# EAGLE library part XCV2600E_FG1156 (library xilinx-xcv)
xcv2600e_fg1156 edit this description Auto generated by make-symbol-device-package-bsdl.ulp Rev. 26 Source: xcv2600e_fg1156.bsd
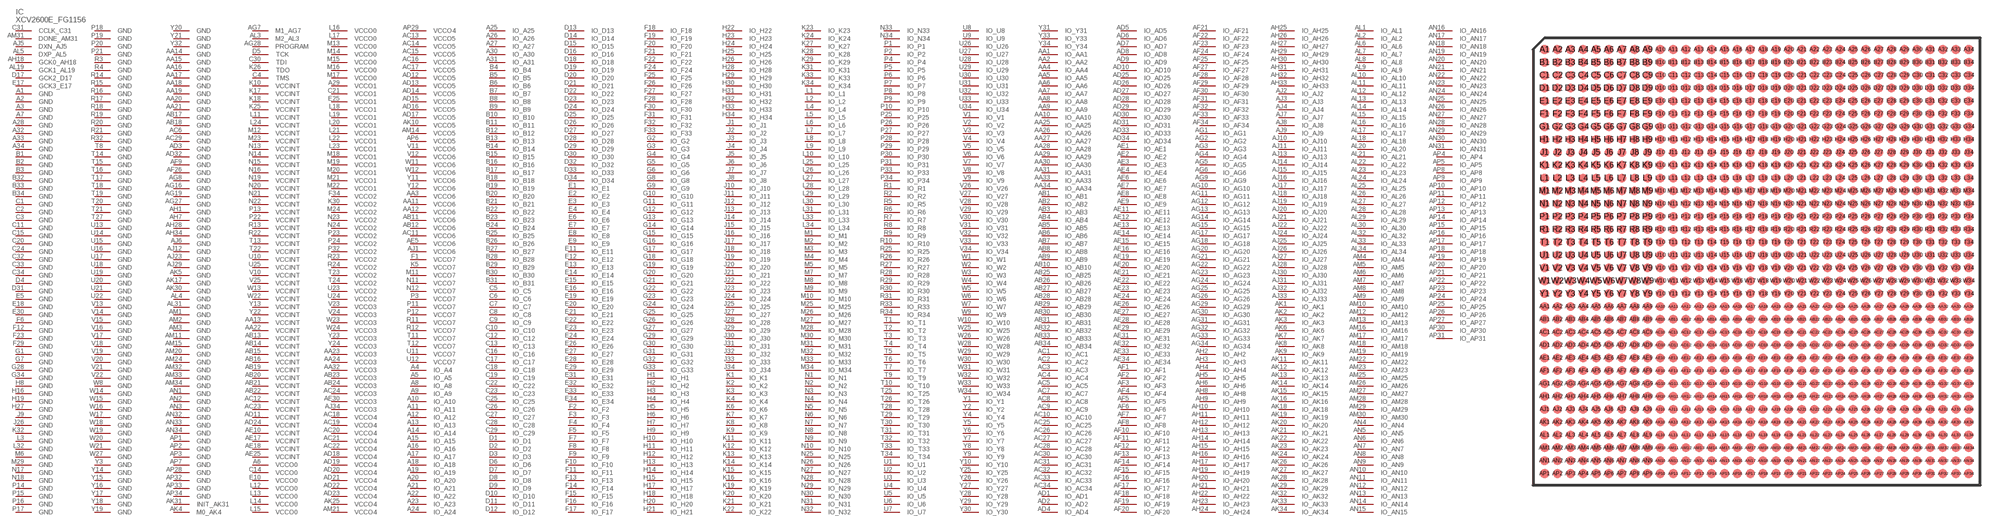
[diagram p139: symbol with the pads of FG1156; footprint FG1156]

Designator prefix IC

## XCV2600E_FG1156 (OC_FARNELL: unknown; OC_NEWARK: unknown)  [FG1156]
A1  GND  pwr
A2  GND  pwr
A3  GND  pwr
A4  IO_A4
A5  IO_A5
A6  VCCO0  pwr
A7  GND  pwr
A8  IO_A8
A9  IO_A9
A10  IO_A10
A11  IO_A11
A12  IO_A12
A13  IO_A13
A14  IO_A14
A15  IO_A15
A16  IO_A16
A17  IO_A17
A18  IO_A18
A19  IO_A19
A20  IO_A20
A21  IO_A21
A22  IO_A22
A23  IO_A23
A24  IO_A24
A25  IO_A25
A26  IO_A26
A27  IO_A27
A28  GND  pwr
A29  VCCO1  pwr
A30  IO_A30
A31  IO_A31
A32  GND  pwr
A33  GND  pwr
A34  GND  pwr
AA1  IO_AA1
AA2  IO_AA2
AA3  VCCO6  pwr
AA4  IO_AA4
AA5  IO_AA5
AA6  IO_AA6
AA7  IO_AA7
AA8  IO_AA8
AA9  IO_AA9
AA10  IO_AA10
AA11  VCCO6  pwr
AA12  VCCO6  pwr
AA13  VCCINT  pwr
AA14  GND  pwr
AA15  GND  pwr
AA16  GND  pwr
AA17  GND  pwr
AA18  GND  pwr
AA19  GND  pwr
AA20  GND  pwr
AA21  GND  pwr
AA22  VCCINT  pwr
AA23  VCCO3  pwr
AA24  VCCO3  pwr
AA25  IO_AA25
AA26  IO_AA26
AA27  IO_AA27
AA28  IO_AA28
AA29  IO_AA29
AA30  IO_AA30
AA31  IO_AA31
AA32  VCCO3  pwr
AA33  IO_AA33
AA34  IO_AA34
AB1  IO_AB1
AB2  IO_AB2
AB3  IO_AB3
AB4  IO_AB4
AB5  IO_AB5
AB6  IO_AB6
AB7  IO_AB7
AB8  IO_AB8
AB9  IO_AB9
AB10  IO_AB10
AB11  VCCO6  pwr
AB12  VCCO6  pwr
AB13  VCCINT  pwr
AB14  VCCINT  pwr
AB15  VCCINT  pwr
AB16  VCCINT  pwr
AB17  GND  pwr
AB18  GND  pwr
AB19  VCCINT  pwr
AB20  VCCINT  pwr
AB21  VCCINT  pwr
AB22  VCCINT  pwr
AB23  VCCO3  pwr
AB24  VCCO3  pwr
AB25  IO_AB25
AB26  IO_AB26
AB27  IO_AB27
AB28  IO_AB28
AB29  IO_AB29
AB30  IO_AB30
AB31  IO_AB31
AB32  IO_AB32
AB33  IO_AB33
AB34  IO_AB34
AC1  IO_AC1
AC2  IO_AC2
AC3  IO_AC3
AC4  IO_AC4
AC5  IO_AC5
AC6  GND  pwr
AC7  IO_AC7
AC8  IO_AC8
AC9  IO_AC9
AC10  IO_AC10
AC11  VCCO6  pwr
AC12  VCCINT  pwr
AC13  VCCO5  pwr
AC14  VCCO5  pwr
AC15  VCCO5  pwr
AC16  VCCO5  pwr
AC17  VCCO5  pwr
AC18  VCCO4  pwr
AC19  VCCO4  pwr
AC20  VCCO4  pwr
AC21  VCCO4  pwr
AC22  VCCO4  pwr
AC23  VCCINT  pwr
AC24  VCCO3  pwr
AC25  IO_AC25
AC26  IO_AC26
AC27  IO_AC27
AC28  IO_AC28
AC29  GND  pwr
AC30  IO_AC30
AC31  IO_AC31
AC32  IO_AC32
AC33  IO_AC33
AC34  IO_AC34
AD1  IO_AD1
AD2  IO_AD2
AD3  GND  pwr
AD4  IO_AD4
AD5  IO_AD5
AD6  IO_AD6
AD7  IO_AD7
AD8  IO_AD8
AD9  IO_AD9
AD10  IO_AD10
AD11  VCCINT  pwr
AD12  VCCO5  pwr
AD13  VCCO5  pwr
AD14  VCCO5  pwr
AD15  VCCO5  pwr
AD16  VCCO5  pwr
AD17  VCCO5  pwr
AD18  VCCO4  pwr
AD19  VCCO4  pwr
AD20  VCCO4  pwr
AD21  VCCO4  pwr
AD22  VCCO4  pwr
AD23  VCCO4  pwr
AD24  VCCINT  pwr
AD25  IO_AD25
AD26  IO_AD26
AD27  IO_AD27
AD28  IO_AD28
AD29  IO_AD29
AD30  IO_AD30
AD31  IO_AD31
AD32  GND  pwr
AD33  IO_AD33
AD34  IO_AD34
AE1  IO_AE1
AE2  IO_AE2
AE3  IO_AE3
AE4  IO_AE4
AE5  VCCO6  pwr
AE6  IO_AE6
AE7  IO_AE7
AE8  IO_AE8
AE9  IO_AE9
AE10  VCCINT  pwr
AE11  IO_AE11
AE12  IO_AE12
AE13  IO_AE13
AE14  IO_AE14
AE15  IO_AE15
AE16  IO_AE16
AE17  VCCINT  pwr
AE18  VCCINT  pwr
AE19  IO_AE19
AE20  IO_AE20
AE21  IO_AE21
AE22  IO_AE22
AE23  IO_AE23
AE24  IO_AE24
AE25  VCCINT  pwr
AE26  IO_AE26
AE27  IO_AE27
AE28  IO_AE28
AE29  IO_AE29
AE30  VCCO3  pwr
AE31  IO_AE31
AE32  IO_AE32
AE33  IO_AE33
AE34  IO_AE34
AF1  IO_AF1
AF2  IO_AF2
AF3  IO_AF3
AF4  IO_AF4
AF5  IO_AF5
AF6  IO_AF6
AF7  IO_AF7
AF8  IO_AF8
AF9  GND  pwr
AF10  IO_AF10
AF11  IO_AF11
AF12  IO_AF12
AF13  IO_AF13
AF14  IO_AF14
AF15  IO_AF15
AF16  IO_AF16
AF17  IO_AF17
AF18  IO_AF18
AF19  IO_AF19
AF20  IO_AF20
AF21  IO_AF21
AF22  IO_AF22
AF23  IO_AF23
AF24  IO_AF24
AF25  IO_AF25
AF26  GND  pwr
AF27  IO_AF27
AF28  IO_AF28
AF29  IO_AF29
AF30  IO_AF30
AF31  IO_AF31
AF32  IO_AF32
AF33  IO_AF33
AF34  IO_AF34
AG1  IO_AG1
AG2  IO_AG2
AG3  IO_AG3
AG4  IO_AG4
AG5  IO_AG5
AG6  IO_AG6
AG7  M1_AG7  in
AG8  GND  pwr
AG9  IO_AG9
AG10  IO_AG10
AG11  IO_AG11
AG12  IO_AG12
AG13  IO_AG13
AG14  IO_AG14
AG15  IO_AG15
AG16  GND  pwr
AG17  IO_AG17
AG18  IO_AG18
AG19  GND  pwr
AG20  IO_AG20
AG21  IO_AG21
AG22  IO_AG22
AG23  IO_AG23
AG24  IO_AG24
AG25  IO_AG25
AG26  IO_AG26
AG27  GND  pwr
AG28  PROGRAM  in
AG29  IO_AG29
AG30  IO_AG30
AG31  IO_AG31
AG32  IO_AG32
AG33  IO_AG33
AG34  IO_AG34
AH1  GND  pwr
AH2  IO_AH2
AH3  IO_AH3
AH4  IO_AH4
AH5  IO_AH5
AH6  IO_AH6
AH7  GND  pwr
AH8  IO_AH8
AH9  IO_AH9
AH10  IO_AH10
AH11  IO_AH11
AH12  IO_AH12
AH13  IO_AH13
AH14  IO_AH14
AH15  IO_AH15
AH16  IO_AH16
AH17  IO_AH17
AH18  GCK0_AH18  in
AH19  IO_AH19
AH20  IO_AH20
AH21  IO_AH21
AH22  IO_AH22
AH23  IO_AH23
AH24  IO_AH24
AH25  IO_AH25
AH26  IO_AH26
AH27  IO_AH27
AH28  GND  pwr
AH29  IO_AH29
AH30  IO_AH30
AH31  IO_AH31
AH32  IO_AH32
AH33  IO_AH33
AH34  GND  pwr
AJ1  VCCO6  pwr
AJ2  IO_AJ2
AJ3  IO_AJ3
AJ4  IO_AJ4
AJ5  DXN_AJ5  pas
AJ6  GND  pwr
AJ7  IO_AJ7
AJ8  IO_AJ8
AJ9  IO_AJ9
AJ10  IO_AJ10
AJ11  IO_AJ11
AJ12  GND  pwr
AJ13  IO_AJ13
AJ14  IO_AJ14
AJ15  IO_AJ15
AJ16  IO_AJ16
AJ17  IO_AJ17
AJ18  IO_AJ18
AJ19  IO_AJ19
AJ20  IO_AJ20
AJ21  IO_AJ21
AJ22  IO_AJ22
AJ23  GND  pwr
AJ24  IO_AJ24
AJ25  IO_AJ25
AJ26  IO_AJ26
AJ27  IO_AJ27
AJ28  IO_AJ28
AJ29  GND  pwr
AJ30  IO_AJ30
AJ31  IO_AJ31
AJ32  IO_AJ32
AJ33  IO_AJ33
AJ34  VCCO3  pwr
AK1  IO_AK1
AK2  IO_AK2
AK3  IO_AK3
AK4  M0_AK4  in
AK5  GND  pwr
AK6  IO_AK6
AK7  IO_AK7
AK8  IO_AK8
AK9  IO_AK9
AK10  VCCO5  pwr
AK11  IO_AK11
AK12  IO_AK12
AK13  IO_AK13
AK14  IO_AK14
AK15  IO_AK15
AK16  IO_AK16
AK17  GND  pwr
AK18  IO_AK18
AK19  IO_AK19
AK20  IO_AK20
AK21  IO_AK21
AK22  IO_AK22
AK23  IO_AK23
AK24  IO_AK24
AK25  VCCO4  pwr
AK26  IO_AK26
AK27  IO_AK27
AK28  IO_AK28
AK29  IO_AK29
AK30  GND  pwr
AK31  INIT_AK31
AK32  IO_AK32
AK33  IO_AK33
AK34  IO_AK34
AL1  IO_AL1
AL2  IO_AL2
AL3  M2_AL3  in
AL4  GND  pwr
AL5  DXP_AL5  pas
AL6  IO_AL6
AL7  IO_AL7
AL8  IO_AL8
AL9  IO_AL9
AL10  IO_AL10
AL11  IO_AL11
AL12  IO_AL12
AL13  IO_AL13
AL14  IO_AL14
AL15  IO_AL15
AL16  IO_AL16
AL17  IO_AL17
AL18  IO_AL18
AL19  GCK1_AL19  in
AL20  IO_AL20
AL21  IO_AL21
AL22  IO_AL22
AL23  IO_AL23
AL24  IO_AL24
AL25  IO_AL25
AL26  IO_AL26
AL27  IO_AL27
AL28  IO_AL28
AL29  IO_AL29
AL30  IO_AL30
AL31  GND  pwr
AL32  IO_AL32
AL33  IO_AL33
AL34  IO_AL34
AM1  GND  pwr
AM2  GND  pwr
AM3  GND  pwr
AM4  IO_AM4
AM5  IO_AM5
AM6  IO_AM6
AM7  IO_AM7
AM8  IO_AM8
AM9  IO_AM9
AM10  IO_AM10
AM11  GND  pwr
AM12  IO_AM12
AM13  IO_AM13
AM14  VCCO5  pwr
AM15  GND  pwr
AM16  IO_AM16
AM17  IO_AM17
AM18  IO_AM18
AM19  IO_AM19
AM20  GND  pwr
AM21  VCCO4  pwr
AM22  IO_AM22
AM23  IO_AM23
AM24  GND  pwr
AM25  IO_AM25
AM26  IO_AM26
AM27  IO_AM27
AM28  IO_AM28
AM29  IO_AM29
AM30  IO_AM30
AM31  DONE_AM31
AM32  GND  pwr
AM33  GND  pwr
AM34  GND  pwr
AN1  GND  pwr
AN2  GND  pwr
AN3  GND  pwr
AN4  IO_AN4
AN5  IO_AN5
AN6  IO_AN6
AN7  IO_AN7
AN8  IO_AN8
AN9  IO_AN9
AN10  IO_AN10
AN11  IO_AN11
AN12  IO_AN12
AN13  IO_AN13
AN14  IO_AN14
AN15  IO_AN15
AN16  IO_AN16
AN17  IO_AN17
AN18  IO_AN18
AN19  IO_AN19
AN20  IO_AN20
AN21  IO_AN21
AN22  IO_AN22
AN23  IO_AN23
AN24  IO_AN24
AN25  IO_AN25
AN26  IO_AN26
AN27  IO_AN27
AN28  IO_AN28
AN29  IO_AN29
AN30  IO_AN30
AN31  IO_AN31
AN32  GND  pwr
AN33  GND  pwr
AN34  GND  pwr
AP1  GND  pwr
AP2  GND  pwr
AP3  GND  pwr
AP4  IO_AP4
AP5  IO_AP5
AP6  VCCO5  pwr
AP7  GND  pwr
AP8  IO_AP8
AP9  IO_AP9
AP10  IO_AP10
AP11  IO_AP11
AP12  IO_AP12
AP13  IO_AP13
AP14  IO_AP14
AP15  IO_AP15
AP16  IO_AP16
AP17  IO_AP17
AP18  IO_AP18
AP19  IO_AP19
AP20  IO_AP20
AP21  IO_AP21
AP22  IO_AP22
AP23  IO_AP23
AP24  IO_AP24
AP25  IO_AP25
AP26  IO_AP26
AP27  IO_AP27
AP28  GND  pwr
AP29  VCCO4  pwr
AP30  IO_AP30
AP31  IO_AP31
AP32  GND  pwr
AP33  GND  pwr
AP34  GND  pwr
B1  GND  pwr
B2  GND  pwr
B3  GND  pwr
B4  IO_B4
B5  IO_B5
B6  IO_B6
B7  IO_B7
B8  IO_B8
B9  IO_B9
B10  IO_B10
B11  IO_B11
B12  IO_B12
B13  IO_B13
B14  IO_B14
B15  IO_B15
B16  IO_B16
B17  IO_B17
B18  IO_B18
B19  IO_B19
B20  IO_B20
B21  IO_B21
B22  IO_B22
B23  IO_B23
B24  IO_B24
B25  IO_B25
B26  IO_B26
B27  IO_B27
B28  IO_B28
B29  IO_B29
B30  IO_B30
B31  IO_B31
B32  GND  pwr
B33  GND  pwr
B34  GND  pwr
C1  GND  pwr
C2  GND  pwr
C3  GND  pwr
C4  TMS  in
C5  IO_C5
C6  IO_C6
C7  IO_C7
C8  IO_C8
C9  IO_C9
C10  IO_C10
C11  GND  pwr
C12  IO_C12
C13  IO_C13
C14  VCCO0  pwr
C15  GND  pwr
C16  IO_C16
C17  IO_C17
C18  IO_C18
C19  IO_C19
C20  GND  pwr
C21  VCCO1  pwr
C22  IO_C22
C23  IO_C23
C24  GND  pwr
C25  IO_C25
C26  IO_C26
C27  IO_C27
C28  IO_C28
C29  IO_C29
C30  TDI  in
C31  CCLK_C31
C32  GND  pwr
C33  GND  pwr
C34  GND  pwr
D1  IO_D1
D2  IO_D2
D3  IO_D3
D4  GND  pwr
D5  TCK  in
D6  IO_D6
D7  IO_D7
D8  IO_D8
D9  IO_D9
D10  IO_D10
D11  IO_D11
D12  IO_D12
D13  IO_D13
D14  IO_D14
D15  IO_D15
D16  IO_D16
D17  GCK2_D17  in
D18  IO_D18
D19  IO_D19
D20  IO_D20
D21  IO_D21
D22  IO_D22
D23  IO_D23
D24  IO_D24
D25  IO_D25
D26  IO_D26
D27  IO_D27
D28  IO_D28
D29  IO_D29
D30  IO_D30
D31  GND  pwr
D32  IO_D32
D33  IO_D33
D34  IO_D34
E1  IO_E1
E2  IO_E2
E3  IO_E3
E4  IO_E4
E5  GND  pwr
E6  IO_E6
E7  IO_E7
E8  IO_E8
E9  IO_E9
E10  VCCO0  pwr
E11  IO_E11
E12  IO_E12
E13  IO_E13
E14  IO_E14
E15  IO_E15
E16  IO_E16
E17  GCK3_E17  in
E18  GND  pwr
E19  IO_E19
E20  IO_E20
E21  IO_E21
E22  IO_E22
E23  IO_E23
E24  IO_E24
E25  VCCO1  pwr
E26  IO_E26
E27  IO_E27
E28  IO_E28
E29  IO_E29
E30  GND  pwr
E31  IO_E31
E32  IO_E32
E33  IO_E33
E34  IO_E34
F1  VCCO7  pwr
F2  IO_F2
F3  IO_F3
F4  IO_F4
F5  IO_F5
F6  GND  pwr
F7  IO_F7
F8  IO_F8
F9  IO_F9
F10  IO_F10
F11  IO_F11
F12  GND  pwr
F13  IO_F13
F14  IO_F14
F15  IO_F15
F16  IO_F16
F17  IO_F17
F18  IO_F18
F19  IO_F19
F20  IO_F20
F21  IO_F21
F22  IO_F22
F23  GND  pwr
F24  IO_F24
F25  IO_F25
F26  IO_F26
F27  IO_F27
F28  IO_F28
F29  GND  pwr
F30  IO_F30
F31  IO_F31
F32  IO_F32
F33  IO_F33
F34  VCCO2  pwr
G1  GND  pwr
G2  IO_G2
G3  IO_G3
G4  IO_G4
G5  IO_G5
G6  IO_G6
G7  GND  pwr
G8  IO_G8
G9  IO_G9
G10  IO_G10
G11  IO_G11
G12  IO_G12
G13  IO_G13
G14  IO_G14
G15  IO_G15
G16  IO_G16
G17  IO_G17
G18  IO_G18
G19  IO_G19
G20  IO_G20
G21  IO_G21
G22  IO_G22
G23  IO_G23
G24  IO_G24
G25  IO_G25
G26  IO_G26
G27  IO_G27
G28  GND  pwr
G29  IO_G29
G30  IO_G30
G31  IO_G31
G32  IO_G32
G33  IO_G33
G34  GND  pwr
H1  IO_H1
H2  IO_H2
H3  IO_H3
H4  IO_H4
H5  IO_H5
H6  IO_H6
H7  IO_H7
H8  GND  pwr
H9  IO_H9
H10  IO_H10
H11  IO_H11
H12  IO_H12
H13  IO_H13
H14  IO_H14
H15  IO_H15
H16  GND  pwr
H17  IO_H17
H18  IO_H18
H19  GND  pwr
H20  IO_H20
H21  IO_H21
H22  IO_H22
H23  IO_H23
H24  IO_H24
H25  IO_H25
H26  IO_H26
H27  GND  pwr
H28  IO_H28
H29  IO_H29
H30  IO_H30
H31  IO_H31
H32  IO_H32
H33  IO_H33
H34  IO_H34
J1  IO_J1
J2  IO_J2
J3  IO_J3
J4  IO_J4
J5  IO_J5
J6  IO_J6
J7  IO_J7
J8  IO_J8
J9  GND  pwr
J10  IO_J10
J11  IO_J11
J12  IO_J12
J13  IO_J13
J14  IO_J14
J15  IO_J15
J16  IO_J16
J17  IO_J17
J18  IO_J18
J19  IO_J19
J20  IO_J20
J21  IO_J21
J22  IO_J22
J23  IO_J23
J24  IO_J24
J25  IO_J25
J26  GND  pwr
J27  IO_J27
J28  IO_J28
J29  IO_J29
J30  IO_J30
J31  IO_J31
J32  IO_J32
J33  IO_J33
J34  IO_J34
K1  IO_K1
K2  IO_K2
K3  IO_K3
K4  IO_K4
K5  VCCO7  pwr
K6  IO_K6
K7  IO_K7
K8  IO_K8
K9  IO_K9
K10  VCCINT  pwr
K11  IO_K11
K12  IO_K12
K13  IO_K13
K14  IO_K14
K15  IO_K15
K16  IO_K16
K17  VCCINT  pwr
K18  VCCINT  pwr
K19  IO_K19
K20  IO_K20
K21  IO_K21
K22  IO_K22
K23  IO_K23
K24  IO_K24
K25  VCCINT  pwr
K26  TDO  out
K27  IO_K27
K28  IO_K28
K29  IO_K29
K30  VCCO2  pwr
K31  IO_K31
K32  GND  pwr
K33  IO_K33
K34  IO_K34
L1  IO_L1
L2  IO_L2
L3  GND  pwr
L4  IO_L4
L5  IO_L5
L6  IO_L6
L7  IO_L7
L8  IO_L8
L9  IO_L9
L10  IO_L10
L11  VCCINT  pwr
L12  VCCO0  pwr
L13  VCCO0  pwr
L14  VCCO0  pwr
L15  VCCO0  pwr
L16  VCCO0  pwr
L17  VCCO0  pwr
L18  VCCO1  pwr
L19  VCCO1  pwr
L20  VCCO1  pwr
L21  VCCO1  pwr
L22  VCCO1  pwr
L23  VCCO1  pwr
L24  VCCINT  pwr
L25  IO_L25
L26  IO_L26
L27  IO_L27
L28  IO_L28
L29  IO_L29
L30  IO_L30
L31  IO_L31
L32  GND  pwr
L33  IO_L33
L34  IO_L34
M1  IO_M1
M2  IO_M2
M3  IO_M3
M4  IO_M4
M5  IO_M5
M6  GND  pwr
M7  IO_M7
M8  IO_M8
M9  IO_M9
M10  IO_M10
M11  VCCO7  pwr
M12  VCCINT  pwr
M13  VCCO0  pwr
M14  VCCO0  pwr
M15  VCCO0  pwr
M16  VCCO0  pwr
M17  VCCO0  pwr
M18  VCCO1  pwr
M19  VCCO1  pwr
M20  VCCO1  pwr
M21  VCCO1  pwr
M22  VCCO1  pwr
M23  VCCINT  pwr
M24  VCCO2  pwr
M25  IO_M25
M26  IO_M26
M27  IO_M27
M28  IO_M28
M29  GND  pwr
M30  IO_M30
M31  IO_M31
M32  IO_M32
M33  IO_M33
M34  IO_M34
N1  IO_N1
N2  IO_N2
N3  IO_N3
N4  IO_N4
N5  IO_N5
N6  IO_N6
N7  IO_N7
N8  IO_N8
N9  IO_N9
N10  IO_N10
N11  VCCO7  pwr
N12  VCCO7  pwr
N13  VCCINT  pwr
N14  VCCINT  pwr
N15  VCCINT  pwr
N16  VCCINT  pwr
N17  GND  pwr
N18  GND  pwr
N19  VCCINT  pwr
N20  VCCINT  pwr
N21  VCCINT  pwr
N22  VCCINT  pwr
N23  VCCO2  pwr
N24  VCCO2  pwr
N25  IO_N25
N26  IO_N26
N27  IO_N27
N28  IO_N28
N29  IO_N29
N30  IO_N30
N31  IO_N31
N32  IO_N32
N33  IO_N33
N34  IO_N34
P1  IO_P1
P2  IO_P2
P3  VCCO7  pwr
P4  IO_P4
P5  IO_P5
P6  IO_P6
P7  IO_P7
P8  IO_P8
P9  IO_P9
P10  IO_P10
P11  VCCO7  pwr
P12  VCCO7  pwr
P13  VCCINT  pwr
P14  GND  pwr
P15  GND  pwr
P16  GND  pwr
P17  GND  pwr
P18  GND  pwr
P19  GND  pwr
P20  GND  pwr
P21  GND  pwr
P22  VCCINT  pwr
P23  VCCO2  pwr
P24  VCCO2  pwr
P25  IO_P25
P26  IO_P26
P27  IO_P27
P28  IO_P28
P29  IO_P29
P30  IO_P30
P31  IO_P31
P32  VCCO2  pwr
P33  IO_P33
P34  IO_P34
R1  IO_R1
R2  IO_R2
R3  GND  pwr
R4  GND  pwr
R5  IO_R5
R6  IO_R6
R7  IO_R7
R8  IO_R8
R9  IO_R9
R10  IO_R10
R11  VCCO7  pwr
R12  VCCO7  pwr
R13  VCCINT  pwr
R14  GND  pwr
R15  GND  pwr
R16  GND  pwr
R17  GND  pwr
R18  GND  pwr
R19  GND  pwr
R20  GND  pwr
R21  GND  pwr
R22  VCCINT  pwr
R23  VCCO2  pwr
R24  VCCO2  pwr
R25  IO_R25
R26  IO_R26
R27  IO_R27
R28  IO_R28
R29  IO_R29
R30  IO_R30
R31  IO_R31
R32  GND  pwr
R33  IO_R33
R34  IO_R34
T1  IO_T1
T2  IO_T2
T3  IO_T3
T4  IO_T4
T5  IO_T5
T6  IO_T6
T7  IO_T7
T8  GND  pwr
T9  IO_T9
T10  IO_T10
T11  VCCO7  pwr
T12  VCCO7  pwr
T13  VCCINT  pwr
T14  GND  pwr
T15  GND  pwr
T16  GND  pwr
T17  GND  pwr
T18  GND  pwr
T19  GND  pwr
T20  GND  pwr
T21  GND  pwr
T22  VCCINT  pwr
T23  VCCO2  pwr
T24  VCCO2  pwr
T25  IO_T25
T26  IO_T26
T27  GND  pwr
T28  IO_T28
T29  IO_T29
T30  IO_T30
T31  IO_T31
T32  IO_T32
T33  IO_T33
T34  IO_T34
U1  IO_U1
U2  IO_U2
U3  IO_U3
U4  IO_U4
U5  IO_U5
U6  IO_U6
U7  IO_U7
U8  IO_U8
U9  IO_U9
U10  VCCINT  pwr
U11  VCCO7  pwr
U12  VCCO7  pwr
U13  GND  pwr
U14  GND  pwr
U15  GND  pwr
U16  GND  pwr
U17  GND  pwr
U18  GND  pwr
U19  GND  pwr
U20  GND  pwr
U21  GND  pwr
U22  GND  pwr
U23  VCCO2  pwr
U24  VCCO2  pwr
U25  VCCINT  pwr
U26  IO_U26
U27  IO_U27
U28  IO_U28
U29  IO_U29
U30  IO_U30
U31  IO_U31
U32  IO_U32
U33  IO_U33
U34  IO_U34
V1  IO_V1
V2  IO_V2
V3  IO_V3
V4  IO_V4
V5  IO_V5
V6  IO_V6
V7  IO_V7
V8  IO_V8
V9  IO_V9
V10  VCCINT  pwr
V11  VCCO6  pwr
V12  VCCO6  pwr
V13  GND  pwr
V14  GND  pwr
V15  GND  pwr
V16  GND  pwr
V17  GND  pwr
V18  GND  pwr
V19  GND  pwr
V20  GND  pwr
V21  GND  pwr
V22  GND  pwr
V23  VCCO3  pwr
V24  VCCO3  pwr
V25  VCCINT  pwr
V26  IO_V26
V27  IO_V27
V28  IO_V28
V29  IO_V29
V30  IO_V30
V31  IO_V31
V32  IO_V32
V33  IO_V33
V34  IO_V34
W1  IO_W1
W2  IO_W2
W3  IO_W3
W4  IO_W4
W5  IO_W5
W6  IO_W6
W7  IO_W7
W8  GND  pwr
W9  IO_W9
W10  IO_W10
W11  VCCO6  pwr
W12  VCCO6  pwr
W13  VCCINT  pwr
W14  GND  pwr
W15  GND  pwr
W16  GND  pwr
W17  GND  pwr
W18  GND  pwr
W19  GND  pwr
W20  GND  pwr
W21  GND  pwr
W22  VCCINT  pwr
W23  VCCO3  pwr
W24  VCCO3  pwr
W25  IO_W25
W26  IO_W26
W27  GND  pwr
W28  IO_W28
W29  IO_W29
W30  IO_W30
W31  IO_W31
W32  IO_W32
W33  IO_W33
W34  IO_W34
Y1  IO_Y1
Y2  IO_Y2
Y3  GND  pwr
Y4  IO_Y4
Y5  IO_Y5
Y6  IO_Y6
Y7  IO_Y7
Y8  IO_Y8
Y9  IO_Y9
Y10  IO_Y10
Y11  VCCO6  pwr
Y12  VCCO6  pwr
Y13  VCCINT  pwr
Y14  GND  pwr
Y15  GND  pwr
Y16  GND  pwr
Y17  GND  pwr
Y18  GND  pwr
Y19  GND  pwr
Y20  GND  pwr
Y21  GND  pwr
Y22  VCCINT  pwr
Y23  VCCO3  pwr
Y24  VCCO3  pwr
Y25  IO_Y25
Y26  IO_Y26
Y27  IO_Y27
Y28  IO_Y28
Y29  IO_Y29
Y30  IO_Y30
Y31  IO_Y31
Y32  GND  pwr
Y33  IO_Y33
Y34  IO_Y34

## Footprint FG1156 (pad centres in mm)
xcv1000e_fg1156_1532 edit this description Auto generated by make-symbol-device-package-bsdl.ulp Rev. 26 Source: xcv1000e_fg1156_1532.bsd
smd 0.7 x 0.7: A1 -16.5,16.5; A2 -15.5,16.5; A3 -14.5,16.5; A4 -13.5,16.5; A5 -12.5,16.5; A6 -11.5,16.5; A7 -10.5,16.5; A8 -9.5,16.5; A9 -8.5,16.5; A10 -7.5,16.5; A11 -6.5,16.5; A12 -5.5,16.5; A13 -4.5,16.5; A14 -3.5,16.5; A15 -2.5,16.5; A16 -1.5,16.5; A17 -0.5,16.5; A18 0.5,16.5; A19 1.5,16.5; A20 2.5,16.5; A21 3.5,16.5; A22 4.5,16.5; A23 5.5,16.5; A24 6.5,16.5; A25 7.5,16.5; A26 8.5,16.5; A27 9.5,16.5; A28 10.5,16.5; A29 11.5,16.5; A30 12.5,16.5; A31 13.5,16.5; A32 14.5,16.5; A33 15.5,16.5; A34 16.5,16.5; AA1 -16.5,-3.5; AA2 -15.5,-3.5; AA3 -14.5,-3.5; AA4 -13.5,-3.5; AA5 -12.5,-3.5; AA6 -11.5,-3.5; AA7 -10.5,-3.5; AA8 -9.5,-3.5; AA9 -8.5,-3.5; AA10 -7.5,-3.5; AA11 -6.5,-3.5; AA12 -5.5,-3.5; AA13 -4.5,-3.5; AA14 -3.5,-3.5; AA15 -2.5,-3.5; AA16 -1.5,-3.5; AA17 -0.5,-3.5; AA18 0.5,-3.5; AA19 1.5,-3.5; AA20 2.5,-3.5; AA21 3.5,-3.5; AA22 4.5,-3.5; AA23 5.5,-3.5; AA24 6.5,-3.5; AA25 7.5,-3.5; AA26 8.5,-3.5; AA27 9.5,-3.5; AA28 10.5,-3.5; AA29 11.5,-3.5; AA30 12.5,-3.5; AA31 13.5,-3.5; AA32 14.5,-3.5; AA33 15.5,-3.5; AA34 16.5,-3.5; AB1 -16.5,-4.5; AB2 -15.5,-4.5; AB3 -14.5,-4.5; AB4 -13.5,-4.5; AB5 -12.5,-4.5; AB6 -11.5,-4.5; AB7 -10.5,-4.5; AB8 -9.5,-4.5; AB9 -8.5,-4.5; AB10 -7.5,-4.5; AB11 -6.5,-4.5; AB12 -5.5,-4.5; AB13 -4.5,-4.5; AB14 -3.5,-4.5; AB15 -2.5,-4.5; AB16 -1.5,-4.5; AB17 -0.5,-4.5; AB18 0.5,-4.5; AB19 1.5,-4.5; AB20 2.5,-4.5; AB21 3.5,-4.5; AB22 4.5,-4.5; AB23 5.5,-4.5; AB24 6.5,-4.5; AB25 7.5,-4.5; AB26 8.5,-4.5; AB27 9.5,-4.5; AB28 10.5,-4.5; AB29 11.5,-4.5; AB30 12.5,-4.5; AB31 13.5,-4.5; AB32 14.5,-4.5; AB33 15.5,-4.5; AB34 16.5,-4.5; AC1 -16.5,-5.5; AC2 -15.5,-5.5; AC3 -14.5,-5.5; AC4 -13.5,-5.5; AC5 -12.5,-5.5; AC6 -11.5,-5.5; AC7 -10.5,-5.5; AC8 -9.5,-5.5; AC9 -8.5,-5.5; AC10 -7.5,-5.5; AC11 -6.5,-5.5; AC12 -5.5,-5.5; AC13 -4.5,-5.5; AC14 -3.5,-5.5; AC15 -2.5,-5.5; AC16 -1.5,-5.5; AC17 -0.5,-5.5; AC18 0.5,-5.5; AC19 1.5,-5.5; AC20 2.5,-5.5; AC21 3.5,-5.5; AC22 4.5,-5.5; AC23 5.5,-5.5; AC24 6.5,-5.5; AC25 7.5,-5.5; AC26 8.5,-5.5; AC27 9.5,-5.5; AC28 10.5,-5.5; AC29 11.5,-5.5; AC30 12.5,-5.5; AC31 13.5,-5.5; AC32 14.5,-5.5; AC33 15.5,-5.5; AC34 16.5,-5.5; AD1 -16.5,-6.5; AD2 -15.5,-6.5; AD3 -14.5,-6.5; AD4 -13.5,-6.5; AD5 -12.5,-6.5; AD6 -11.5,-6.5; AD7 -10.5,-6.5; AD8 -9.5,-6.5; AD9 -8.5,-6.5; AD10 -7.5,-6.5; AD11 -6.5,-6.5; AD12 -5.5,-6.5; AD13 -4.5,-6.5; AD14 -3.5,-6.5; AD15 -2.5,-6.5; AD16 -1.5,-6.5; AD17 -0.5,-6.5; AD18 0.5,-6.5; AD19 1.5,-6.5; AD20 2.5,-6.5; AD21 3.5,-6.5; AD22 4.5,-6.5; AD23 5.5,-6.5; AD24 6.5,-6.5; AD25 7.5,-6.5; AD26 8.5,-6.5; AD27 9.5,-6.5; AD28 10.5,-6.5; AD29 11.5,-6.5; AD30 12.5,-6.5; AD31 13.5,-6.5; AD32 14.5,-6.5; AD33 15.5,-6.5; AD34 16.5,-6.5; AE1 -16.5,-7.5; AE2 -15.5,-7.5; AE3 -14.5,-7.5; AE4 -13.5,-7.5; AE5 -12.5,-7.5; AE6 -11.5,-7.5; AE7 -10.5,-7.5; AE8 -9.5,-7.5; AE9 -8.5,-7.5; AE10 -7.5,-7.5; AE11 -6.5,-7.5; AE12 -5.5,-7.5; AE13 -4.5,-7.5; AE14 -3.5,-7.5; AE15 -2.5,-7.5; AE16 -1.5,-7.5; AE17 -0.5,-7.5; AE18 0.5,-7.5; AE19 1.5,-7.5; AE20 2.5,-7.5; AE21 3.5,-7.5; AE22 4.5,-7.5; AE23 5.5,-7.5; AE24 6.5,-7.5; AE25 7.5,-7.5; AE26 8.5,-7.5; AE27 9.5,-7.5; AE28 10.5,-7.5; AE29 11.5,-7.5; AE30 12.5,-7.5; AE31 13.5,-7.5; AE32 14.5,-7.5; AE33 15.5,-7.5; AE34 16.5,-7.5; AF1 -16.5,-8.5; AF2 -15.5,-8.5; AF3 -14.5,-8.5; AF4 -13.5,-8.5; AF5 -12.5,-8.5; AF6 -11.5,-8.5; AF7 -10.5,-8.5; AF8 -9.5,-8.5; AF9 -8.5,-8.5; AF10 -7.5,-8.5; AF11 -6.5,-8.5; AF12 -5.5,-8.5; AF13 -4.5,-8.5; AF14 -3.5,-8.5; AF15 -2.5,-8.5; AF16 -1.5,-8.5; AF17 -0.5,-8.5; AF18 0.5,-8.5; AF19 1.5,-8.5; AF20 2.5,-8.5; AF21 3.5,-8.5; AF22 4.5,-8.5; AF23 5.5,-8.5; AF24 6.5,-8.5; AF25 7.5,-8.5; AF26 8.5,-8.5; AF27 9.5,-8.5; AF28 10.5,-8.5; AF29 11.5,-8.5; AF30 12.5,-8.5; AF31 13.5,-8.5; AF32 14.5,-8.5; AF33 15.5,-8.5; AF34 16.5,-8.5; AG1 -16.5,-9.5; AG2 -15.5,-9.5; AG3 -14.5,-9.5; AG4 -13.5,-9.5; AG5 -12.5,-9.5; AG6 -11.5,-9.5; AG7 -10.5,-9.5; AG8 -9.5,-9.5; AG9 -8.5,-9.5; AG10 -7.5,-9.5; AG11 -6.5,-9.5; AG12 -5.5,-9.5; AG13 -4.5,-9.5; AG14 -3.5,-9.5; AG15 -2.5,-9.5; AG16 -1.5,-9.5; AG17 -0.5,-9.5; AG18 0.5,-9.5; AG19 1.5,-9.5; AG20 2.5,-9.5; AG21 3.5,-9.5; AG22 4.5,-9.5; AG23 5.5,-9.5; AG24 6.5,-9.5; AG25 7.5,-9.5; AG26 8.5,-9.5; AG27 9.5,-9.5; AG28 10.5,-9.5; AG29 11.5,-9.5; AG30 12.5,-9.5; AG31 13.5,-9.5; AG32 14.5,-9.5; AG33 15.5,-9.5; AG34 16.5,-9.5; AH1 -16.5,-10.5; AH2 -15.5,-10.5; AH3 -14.5,-10.5; AH4 -13.5,-10.5; AH5 -12.5,-10.5; AH6 -11.5,-10.5; AH7 -10.5,-10.5; AH8 -9.5,-10.5; AH9 -8.5,-10.5; AH10 -7.5,-10.5; AH11 -6.5,-10.5; AH12 -5.5,-10.5; AH13 -4.5,-10.5; AH14 -3.5,-10.5; AH15 -2.5,-10.5; AH16 -1.5,-10.5; AH17 -0.5,-10.5; AH18 0.5,-10.5; AH19 1.5,-10.5; AH20 2.5,-10.5; AH21 3.5,-10.5; AH22 4.5,-10.5; AH23 5.5,-10.5; AH24 6.5,-10.5; AH25 7.5,-10.5; AH26 8.5,-10.5; AH27 9.5,-10.5; AH28 10.5,-10.5; AH29 11.5,-10.5; AH30 12.5,-10.5; AH31 13.5,-10.5; AH32 14.5,-10.5; AH33 15.5,-10.5; AH34 16.5,-10.5; AJ1 -16.5,-11.5; AJ2 -15.5,-11.5; AJ3 -14.5,-11.5; AJ4 -13.5,-11.5; AJ5 -12.5,-11.5; AJ6 -11.5,-11.5; AJ7 -10.5,-11.5; AJ8 -9.5,-11.5; AJ9 -8.5,-11.5; AJ10 -7.5,-11.5; AJ11 -6.5,-11.5; AJ12 -5.5,-11.5; AJ13 -4.5,-11.5; AJ14 -3.5,-11.5; AJ15 -2.5,-11.5; AJ16 -1.5,-11.5; AJ17 -0.5,-11.5; AJ18 0.5,-11.5; AJ19 1.5,-11.5; AJ20 2.5,-11.5; AJ21 3.5,-11.5; AJ22 4.5,-11.5; AJ23 5.5,-11.5; AJ24 6.5,-11.5; AJ25 7.5,-11.5; AJ26 8.5,-11.5; AJ27 9.5,-11.5; AJ28 10.5,-11.5; AJ29 11.5,-11.5; AJ30 12.5,-11.5; AJ31 13.5,-11.5; AJ32 14.5,-11.5; AJ33 15.5,-11.5; AJ34 16.5,-11.5; AK1 -16.5,-12.5; AK2 -15.5,-12.5; AK3 -14.5,-12.5; AK4 -13.5,-12.5; AK5 -12.5,-12.5; AK6 -11.5,-12.5; AK7 -10.5,-12.5; AK8 -9.5,-12.5; AK9 -8.5,-12.5; AK10 -7.5,-12.5; AK11 -6.5,-12.5; AK12 -5.5,-12.5; AK13 -4.5,-12.5; AK14 -3.5,-12.5; AK15 -2.5,-12.5; AK16 -1.5,-12.5; AK17 -0.5,-12.5; AK18 0.5,-12.5; AK19 1.5,-12.5; AK20 2.5,-12.5; AK21 3.5,-12.5; AK22 4.5,-12.5; AK23 5.5,-12.5; AK24 6.5,-12.5; AK25 7.5,-12.5; AK26 8.5,-12.5; AK27 9.5,-12.5; AK28 10.5,-12.5; AK29 11.5,-12.5; AK30 12.5,-12.5; AK31 13.5,-12.5; AK32 14.5,-12.5; AK33 15.5,-12.5; AK34 16.5,-12.5; AL1 -16.5,-13.5; AL2 -15.5,-13.5; AL3 -14.5,-13.5; AL4 -13.5,-13.5; AL5 -12.5,-13.5; AL6 -11.5,-13.5; AL7 -10.5,-13.5; AL8 -9.5,-13.5; AL9 -8.5,-13.5; AL10 -7.5,-13.5; AL11 -6.5,-13.5; AL12 -5.5,-13.5; AL13 -4.5,-13.5; AL14 -3.5,-13.5; AL15 -2.5,-13.5; AL16 -1.5,-13.5; AL17 -0.5,-13.5; AL18 0.5,-13.5; AL19 1.5,-13.5; AL20 2.5,-13.5; AL21 3.5,-13.5; AL22 4.5,-13.5; AL23 5.5,-13.5; AL24 6.5,-13.5; AL25 7.5,-13.5; AL26 8.5,-13.5; AL27 9.5,-13.5; AL28 10.5,-13.5; AL29 11.5,-13.5; AL30 12.5,-13.5; AL31 13.5,-13.5; AL32 14.5,-13.5; AL33 15.5,-13.5; AL34 16.5,-13.5; AM1 -16.5,-14.5; AM2 -15.5,-14.5; AM3 -14.5,-14.5; AM4 -13.5,-14.5; AM5 -12.5,-14.5; AM6 -11.5,-14.5; AM7 -10.5,-14.5; AM8 -9.5,-14.5; AM9 -8.5,-14.5; AM10 -7.5,-14.5; AM11 -6.5,-14.5; AM12 -5.5,-14.5; AM13 -4.5,-14.5; AM14 -3.5,-14.5; AM15 -2.5,-14.5; AM16 -1.5,-14.5; AM17 -0.5,-14.5; AM18 0.5,-14.5; AM19 1.5,-14.5; AM20 2.5,-14.5; AM21 3.5,-14.5; AM22 4.5,-14.5; AM23 5.5,-14.5; AM24 6.5,-14.5; AM25 7.5,-14.5; AM26 8.5,-14.5; AM27 9.5,-14.5; AM28 10.5,-14.5; AM29 11.5,-14.5; AM30 12.5,-14.5; AM31 13.5,-14.5; AM32 14.5,-14.5; AM33 15.5,-14.5; AM34 16.5,-14.5; AN1 -16.5,-15.5; AN2 -15.5,-15.5; AN3 -14.5,-15.5; AN4 -13.5,-15.5; AN5 -12.5,-15.5; AN6 -11.5,-15.5; AN7 -10.5,-15.5; AN8 -9.5,-15.5; AN9 -8.5,-15.5; AN10 -7.5,-15.5; AN11 -6.5,-15.5; AN12 -5.5,-15.5; AN13 -4.5,-15.5; AN14 -3.5,-15.5; AN15 -2.5,-15.5; AN16 -1.5,-15.5; AN17 -0.5,-15.5; AN18 0.5,-15.5; AN19 1.5,-15.5; AN20 2.5,-15.5; AN21 3.5,-15.5; AN22 4.5,-15.5; AN23 5.5,-15.5; AN24 6.5,-15.5; AN25 7.5,-15.5; AN26 8.5,-15.5; AN27 9.5,-15.5; AN28 10.5,-15.5; AN29 11.5,-15.5; AN30 12.5,-15.5; AN31 13.5,-15.5; AN32 14.5,-15.5; AN33 15.5,-15.5; AN34 16.5,-15.5; AP1 -16.5,-16.5; AP2 -15.5,-16.5; AP3 -14.5,-16.5; AP4 -13.5,-16.5; AP5 -12.5,-16.5; AP6 -11.5,-16.5; AP7 -10.5,-16.5; AP8 -9.5,-16.5; AP9 -8.5,-16.5; AP10 -7.5,-16.5; AP11 -6.5,-16.5; AP12 -5.5,-16.5; AP13 -4.5,-16.5; AP14 -3.5,-16.5; AP15 -2.5,-16.5; AP16 -1.5,-16.5; AP17 -0.5,-16.5; AP18 0.5,-16.5; AP19 1.5,-16.5; AP20 2.5,-16.5; AP21 3.5,-16.5; AP22 4.5,-16.5; AP23 5.5,-16.5; AP24 6.5,-16.5; AP25 7.5,-16.5; AP26 8.5,-16.5; AP27 9.5,-16.5; AP28 10.5,-16.5; AP29 11.5,-16.5; AP30 12.5,-16.5; AP31 13.5,-16.5; AP32 14.5,-16.5; AP33 15.5,-16.5; AP34 16.5,-16.5; B1 -16.5,15.5; B2 -15.5,15.5; B3 -14.5,15.5; B4 -13.5,15.5; B5 -12.5,15.5; B6 -11.5,15.5; B7 -10.5,15.5; B8 -9.5,15.5; B9 -8.5,15.5; B10 -7.5,15.5; B11 -6.5,15.5; B12 -5.5,15.5; B13 -4.5,15.5; B14 -3.5,15.5; B15 -2.5,15.5; B16 -1.5,15.5; B17 -0.5,15.5; B18 0.5,15.5; B19 1.5,15.5; B20 2.5,15.5; B21 3.5,15.5; B22 4.5,15.5; B23 5.5,15.5; B24 6.5,15.5; B25 7.5,15.5; B26 8.5,15.5; B27 9.5,15.5; B28 10.5,15.5; B29 11.5,15.5; B30 12.5,15.5; B31 13.5,15.5; B32 14.5,15.5; B33 15.5,15.5; B34 16.5,15.5; C1 -16.5,14.5; C2 -15.5,14.5; C3 -14.5,14.5; C4 -13.5,14.5; C5 -12.5,14.5; C6 -11.5,14.5; C7 -10.5,14.5; C8 -9.5,14.5; C9 -8.5,14.5; C10 -7.5,14.5; C11 -6.5,14.5; C12 -5.5,14.5; C13 -4.5,14.5; C14 -3.5,14.5; C15 -2.5,14.5; C16 -1.5,14.5; C17 -0.5,14.5; C18 0.5,14.5; C19 1.5,14.5; C20 2.5,14.5; C21 3.5,14.5; C22 4.5,14.5; C23 5.5,14.5; C24 6.5,14.5; C25 7.5,14.5; C26 8.5,14.5; C27 9.5,14.5; C28 10.5,14.5; C29 11.5,14.5; C30 12.5,14.5; C31 13.5,14.5; C32 14.5,14.5; C33 15.5,14.5; C34 16.5,14.5; D1 -16.5,13.5; D2 -15.5,13.5; D3 -14.5,13.5; D4 -13.5,13.5; D5 -12.5,13.5; D6 -11.5,13.5; D7 -10.5,13.5; D8 -9.5,13.5; D9 -8.5,13.5; D10 -7.5,13.5; D11 -6.5,13.5; D12 -5.5,13.5; D13 -4.5,13.5; D14 -3.5,13.5; D15 -2.5,13.5; D16 -1.5,13.5; D17 -0.5,13.5; D18 0.5,13.5; D19 1.5,13.5; D20 2.5,13.5; D21 3.5,13.5; D22 4.5,13.5; D23 5.5,13.5; D24 6.5,13.5; D25 7.5,13.5; D26 8.5,13.5; D27 9.5,13.5; D28 10.5,13.5; D29 11.5,13.5; D30 12.5,13.5; D31 13.5,13.5; D32 14.5,13.5; D33 15.5,13.5; D34 16.5,13.5; E1 -16.5,12.5; E2 -15.5,12.5; E3 -14.5,12.5; E4 -13.5,12.5; E5 -12.5,12.5; E6 -11.5,12.5; E7 -10.5,12.5; E8 -9.5,12.5; E9 -8.5,12.5; E10 -7.5,12.5; E11 -6.5,12.5; E12 -5.5,12.5; E13 -4.5,12.5; E14 -3.5,12.5; E15 -2.5,12.5; E16 -1.5,12.5; E17 -0.5,12.5; E18 0.5,12.5; E19 1.5,12.5; E20 2.5,12.5; E21 3.5,12.5; E22 4.5,12.5; E23 5.5,12.5; E24 6.5,12.5; E25 7.5,12.5; E26 8.5,12.5; E27 9.5,12.5; E28 10.5,12.5; E29 11.5,12.5; E30 12.5,12.5; E31 13.5,12.5; E32 14.5,12.5; E33 15.5,12.5; E34 16.5,12.5; F1 -16.5,11.5; F2 -15.5,11.5; F3 -14.5,11.5; F4 -13.5,11.5; F5 -12.5,11.5; F6 -11.5,11.5; F7 -10.5,11.5; F8 -9.5,11.5; F9 -8.5,11.5; F10 -7.5,11.5; F11 -6.5,11.5; F12 -5.5,11.5; F13 -4.5,11.5; F14 -3.5,11.5; F15 -2.5,11.5; F16 -1.5,11.5; F17 -0.5,11.5; F18 0.5,11.5; F19 1.5,11.5; F20 2.5,11.5; F21 3.5,11.5; F22 4.5,11.5; F23 5.5,11.5; F24 6.5,11.5; F25 7.5,11.5; F26 8.5,11.5; F27 9.5,11.5; F28 10.5,11.5; F29 11.5,11.5; F30 12.5,11.5; F31 13.5,11.5; F32 14.5,11.5; F33 15.5,11.5; F34 16.5,11.5; G1 -16.5,10.5; G2 -15.5,10.5; G3 -14.5,10.5; G4 -13.5,10.5; G5 -12.5,10.5; G6 -11.5,10.5; G7 -10.5,10.5; G8 -9.5,10.5; G9 -8.5,10.5; G10 -7.5,10.5; G11 -6.5,10.5; G12 -5.5,10.5; G13 -4.5,10.5; G14 -3.5,10.5; G15 -2.5,10.5; G16 -1.5,10.5; G17 -0.5,10.5; G18 0.5,10.5; G19 1.5,10.5; G20 2.5,10.5; G21 3.5,10.5; G22 4.5,10.5; G23 5.5,10.5; G24 6.5,10.5; G25 7.5,10.5; G26 8.5,10.5; G27 9.5,10.5; G28 10.5,10.5; G29 11.5,10.5; G30 12.5,10.5; G31 13.5,10.5; G32 14.5,10.5; G33 15.5,10.5; G34 16.5,10.5; H1 -16.5,9.5; H2 -15.5,9.5; H3 -14.5,9.5; H4 -13.5,9.5; H5 -12.5,9.5; H6 -11.5,9.5; H7 -10.5,9.5; H8 -9.5,9.5; H9 -8.5,9.5; H10 -7.5,9.5; H11 -6.5,9.5; H12 -5.5,9.5; H13 -4.5,9.5; H14 -3.5,9.5; H15 -2.5,9.5; H16 -1.5,9.5; H17 -0.5,9.5; H18 0.5,9.5; H19 1.5,9.5; H20 2.5,9.5; H21 3.5,9.5; H22 4.5,9.5; H23 5.5,9.5; H24 6.5,9.5; H25 7.5,9.5; H26 8.5,9.5; H27 9.5,9.5; H28 10.5,9.5; H29 11.5,9.5; H30 12.5,9.5; H31 13.5,9.5; H32 14.5,9.5; H33 15.5,9.5; H34 16.5,9.5; J1 -16.5,8.5; J2 -15.5,8.5; J3 -14.5,8.5; J4 -13.5,8.5; J5 -12.5,8.5; J6 -11.5,8.5; J7 -10.5,8.5; J8 -9.5,8.5; J9 -8.5,8.5; J10 -7.5,8.5; J11 -6.5,8.5; J12 -5.5,8.5; J13 -4.5,8.5; J14 -3.5,8.5; J15 -2.5,8.5; J16 -1.5,8.5; J17 -0.5,8.5; J18 0.5,8.5; J19 1.5,8.5; J20 2.5,8.5; J21 3.5,8.5; J22 4.5,8.5; J23 5.5,8.5; J24 6.5,8.5; J25 7.5,8.5; J26 8.5,8.5; J27 9.5,8.5; J28 10.5,8.5; J29 11.5,8.5; J30 12.5,8.5; J31 13.5,8.5; J32 14.5,8.5; J33 15.5,8.5; J34 16.5,8.5; K1 -16.5,7.5; K2 -15.5,7.5; K3 -14.5,7.5; K4 -13.5,7.5; K5 -12.5,7.5; K6 -11.5,7.5; K7 -10.5,7.5; K8 -9.5,7.5; K9 -8.5,7.5; K10 -7.5,7.5; K11 -6.5,7.5; K12 -5.5,7.5; K13 -4.5,7.5; K14 -3.5,7.5; K15 -2.5,7.5; K16 -1.5,7.5; K17 -0.5,7.5; K18 0.5,7.5; K19 1.5,7.5; K20 2.5,7.5; K21 3.5,7.5; K22 4.5,7.5; K23 5.5,7.5; K24 6.5,7.5; K25 7.5,7.5; K26 8.5,7.5; K27 9.5,7.5; K28 10.5,7.5; K29 11.5,7.5; K30 12.5,7.5; K31 13.5,7.5; K32 14.5,7.5; K33 15.5,7.5; K34 16.5,7.5; L1 -16.5,6.5; L2 -15.5,6.5; L3 -14.5,6.5; L4 -13.5,6.5; L5 -12.5,6.5; L6 -11.5,6.5; L7 -10.5,6.5; L8 -9.5,6.5; L9 -8.5,6.5; L10 -7.5,6.5; L11 -6.5,6.5; L12 -5.5,6.5; L13 -4.5,6.5; L14 -3.5,6.5; L15 -2.5,6.5; L16 -1.5,6.5; L17 -0.5,6.5; L18 0.5,6.5; L19 1.5,6.5; L20 2.5,6.5; L21 3.5,6.5; L22 4.5,6.5; L23 5.5,6.5; L24 6.5,6.5; L25 7.5,6.5; L26 8.5,6.5; L27 9.5,6.5; L28 10.5,6.5; L29 11.5,6.5; L30 12.5,6.5; L31 13.5,6.5; L32 14.5,6.5; L33 15.5,6.5; L34 16.5,6.5; M1 -16.5,5.5; M2 -15.5,5.5; M3 -14.5,5.5; M4 -13.5,5.5; M5 -12.5,5.5; M6 -11.5,5.5; M7 -10.5,5.5; M8 -9.5,5.5; M9 -8.5,5.5; M10 -7.5,5.5; M11 -6.5,5.5; M12 -5.5,5.5; M13 -4.5,5.5; M14 -3.5,5.5; M15 -2.5,5.5; M16 -1.5,5.5; M17 -0.5,5.5; M18 0.5,5.5; M19 1.5,5.5; M20 2.5,5.5; M21 3.5,5.5; M22 4.5,5.5; M23 5.5,5.5; M24 6.5,5.5; M25 7.5,5.5; M26 8.5,5.5; M27 9.5,5.5; M28 10.5,5.5; M29 11.5,5.5; M30 12.5,5.5; M31 13.5,5.5; M32 14.5,5.5; M33 15.5,5.5; M34 16.5,5.5; N1 -16.5,4.5; N2 -15.5,4.5; N3 -14.5,4.5; N4 -13.5,4.5; N5 -12.5,4.5; N6 -11.5,4.5; N7 -10.5,4.5; N8 -9.5,4.5; N9 -8.5,4.5; N10 -7.5,4.5; N11 -6.5,4.5; N12 -5.5,4.5; N13 -4.5,4.5; N14 -3.5,4.5; N15 -2.5,4.5; N16 -1.5,4.5; N17 -0.5,4.5; N18 0.5,4.5; N19 1.5,4.5; N20 2.5,4.5; N21 3.5,4.5; N22 4.5,4.5; N23 5.5,4.5; N24 6.5,4.5; N25 7.5,4.5; N26 8.5,4.5; N27 9.5,4.5; N28 10.5,4.5; N29 11.5,4.5; N30 12.5,4.5; N31 13.5,4.5; N32 14.5,4.5; N33 15.5,4.5; N34 16.5,4.5; P1 -16.5,3.5; P2 -15.5,3.5; P3 -14.5,3.5; P4 -13.5,3.5; P5 -12.5,3.5; P6 -11.5,3.5; P7 -10.5,3.5; P8 -9.5,3.5; P9 -8.5,3.5; P10 -7.5,3.5; P11 -6.5,3.5; P12 -5.5,3.5; P13 -4.5,3.5; P14 -3.5,3.5; P15 -2.5,3.5; P16 -1.5,3.5; P17 -0.5,3.5; P18 0.5,3.5; P19 1.5,3.5; P20 2.5,3.5; P21 3.5,3.5; P22 4.5,3.5; P23 5.5,3.5; P24 6.5,3.5; P25 7.5,3.5; P26 8.5,3.5; P27 9.5,3.5; P28 10.5,3.5; P29 11.5,3.5; P30 12.5,3.5; P31 13.5,3.5; P32 14.5,3.5; P33 15.5,3.5; P34 16.5,3.5; R1 -16.5,2.5; R2 -15.5,2.5; R3 -14.5,2.5; R4 -13.5,2.5; R5 -12.5,2.5; R6 -11.5,2.5; R7 -10.5,2.5; R8 -9.5,2.5; R9 -8.5,2.5; R10 -7.5,2.5; R11 -6.5,2.5; R12 -5.5,2.5; R13 -4.5,2.5; R14 -3.5,2.5; R15 -2.5,2.5; R16 -1.5,2.5; R17 -0.5,2.5; R18 0.5,2.5; R19 1.5,2.5; R20 2.5,2.5; R21 3.5,2.5; R22 4.5,2.5; R23 5.5,2.5; R24 6.5,2.5; R25 7.5,2.5; R26 8.5,2.5; R27 9.5,2.5; R28 10.5,2.5; R29 11.5,2.5; R30 12.5,2.5; R31 13.5,2.5; R32 14.5,2.5; R33 15.5,2.5; R34 16.5,2.5; T1 -16.5,1.5; T2 -15.5,1.5; T3 -14.5,1.5; T4 -13.5,1.5; T5 -12.5,1.5; T6 -11.5,1.5; T7 -10.5,1.5; T8 -9.5,1.5; T9 -8.5,1.5; T10 -7.5,1.5; T11 -6.5,1.5; T12 -5.5,1.5; T13 -4.5,1.5; T14 -3.5,1.5; T15 -2.5,1.5; T16 -1.5,1.5; T17 -0.5,1.5; T18 0.5,1.5; T19 1.5,1.5; T20 2.5,1.5; T21 3.5,1.5; T22 4.5,1.5; T23 5.5,1.5; T24 6.5,1.5; T25 7.5,1.5; T26 8.5,1.5; T27 9.5,1.5; T28 10.5,1.5; T29 11.5,1.5; T30 12.5,1.5; T31 13.5,1.5; T32 14.5,1.5; T33 15.5,1.5; T34 16.5,1.5; U1 -16.5,0.5; U2 -15.5,0.5; U3 -14.5,0.5; U4 -13.5,0.5; U5 -12.5,0.5; U6 -11.5,0.5; U7 -10.5,0.5; U8 -9.5,0.5; U9 -8.5,0.5; U10 -7.5,0.5; U11 -6.5,0.5; U12 -5.5,0.5; U13 -4.5,0.5; U14 -3.5,0.5; U15 -2.5,0.5; U16 -1.5,0.5; U17 -0.5,0.5; U18 0.5,0.5; U19 1.5,0.5; U20 2.5,0.5; U21 3.5,0.5; U22 4.5,0.5; U23 5.5,0.5; U24 6.5,0.5; U25 7.5,0.5; U26 8.5,0.5; U27 9.5,0.5; U28 10.5,0.5; U29 11.5,0.5; U30 12.5,0.5; U31 13.5,0.5; U32 14.5,0.5; U33 15.5,0.5; U34 16.5,0.5; V1 -16.5,-0.5; V2 -15.5,-0.5; V3 -14.5,-0.5; V4 -13.5,-0.5; V5 -12.5,-0.5; V6 -11.5,-0.5; V7 -10.5,-0.5; V8 -9.5,-0.5; V9 -8.5,-0.5; V10 -7.5,-0.5; V11 -6.5,-0.5; V12 -5.5,-0.5; V13 -4.5,-0.5; V14 -3.5,-0.5; V15 -2.5,-0.5; V16 -1.5,-0.5; V17 -0.5,-0.5; V18 0.5,-0.5; V19 1.5,-0.5; V20 2.5,-0.5; V21 3.5,-0.5; V22 4.5,-0.5; V23 5.5,-0.5; V24 6.5,-0.5; V25 7.5,-0.5; V26 8.5,-0.5; V27 9.5,-0.5; V28 10.5,-0.5; V29 11.5,-0.5; V30 12.5,-0.5; V31 13.5,-0.5; V32 14.5,-0.5; V33 15.5,-0.5; V34 16.5,-0.5; W1 -16.5,-1.5; W2 -15.5,-1.5; W3 -14.5,-1.5; W4 -13.5,-1.5; W5 -12.5,-1.5; W6 -11.5,-1.5; W7 -10.5,-1.5; W8 -9.5,-1.5; W9 -8.5,-1.5; W10 -7.5,-1.5; W11 -6.5,-1.5; W12 -5.5,-1.5; W13 -4.5,-1.5; W14 -3.5,-1.5; W15 -2.5,-1.5; W16 -1.5,-1.5; W17 -0.5,-1.5; W18 0.5,-1.5; W19 1.5,-1.5; W20 2.5,-1.5; W21 3.5,-1.5; W22 4.5,-1.5; W23 5.5,-1.5; W24 6.5,-1.5; W25 7.5,-1.5; W26 8.5,-1.5; W27 9.5,-1.5; W28 10.5,-1.5; W29 11.5,-1.5; W30 12.5,-1.5; W31 13.5,-1.5; W32 14.5,-1.5; W33 15.5,-1.5; W34 16.5,-1.5; Y1 -16.5,-2.5; Y2 -15.5,-2.5; Y3 -14.5,-2.5; Y4 -13.5,-2.5; Y5 -12.5,-2.5; Y6 -11.5,-2.5; Y7 -10.5,-2.5; Y8 -9.5,-2.5; Y9 -8.5,-2.5; Y10 -7.5,-2.5; Y11 -6.5,-2.5; Y12 -5.5,-2.5; Y13 -4.5,-2.5; Y14 -3.5,-2.5; Y15 -2.5,-2.5; Y16 -1.5,-2.5; Y17 -0.5,-2.5; Y18 0.5,-2.5; Y19 1.5,-2.5; Y20 2.5,-2.5; Y21 3.5,-2.5; Y22 4.5,-2.5; Y23 5.5,-2.5; Y24 6.5,-2.5; Y25 7.5,-2.5; Y26 8.5,-2.5; Y27 9.5,-2.5; Y28 10.5,-2.5; Y29 11.5,-2.5; Y30 12.5,-2.5; Y31 13.5,-2.5; Y32 14.5,-2.5; Y33 15.5,-2.5; Y34 16.5,-2.5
